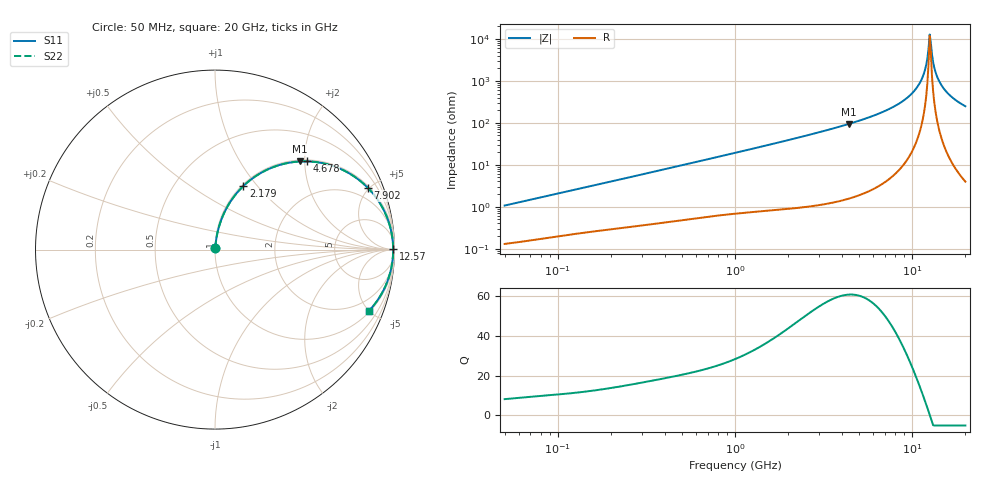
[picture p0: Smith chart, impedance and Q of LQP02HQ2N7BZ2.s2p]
!Murata Part Number: LQP02HQ2N7BZ2
!These Parameters are Measured in Series Mode Connection
!  o--[Z]--o
!Port1  Port2
!  o-------o
!Freq. Start=50[MHz] Stop=20[GHz], 401[Steps]
# Hz S RI R 50
!Freq.(Hz) S11(Real) S11(Imag) S21(Real) S21(Imag) S12(Real) S12(Imag) S22(Real) S22(Imag)
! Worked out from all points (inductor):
!   401 points, 50 MHz to 20 GHz, reference 50 ohm
!   read as one part in series: L = 3.34 nH near 51.52 MHz
!   highest Q = 60.5 at 4.406 GHz (marker M1), where L = 3.41 nH
!   self-resonance near 12.57 GHz
!   S11 on the Smith chart (normalised r, x): 50 MHz: 1.00, +0.02; 2.179 GHz: 1.02, +0.85; 4.678 GHz: 1.03, +2.04; 7.902 GHz: 1.11, +4.89; 12.57 GHz: open; 20 GHz: 1.08, -4.97
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5e7  0.00141 0.0105  0.9986 -0.0105  0.9986 -0.0105  0.00141 0.0105
1.364002e8  0.00311 0.0275  0.9969 -0.0275  0.9969 -0.0275  0.00311 0.0275
3.721004e8  0.00922 0.0718  0.9908 -0.0718  0.9908 -0.0718  0.00922 0.0718
1e9  0.0416 0.1826  0.9584 -0.1826  0.9584 -0.1826  0.0416 0.1826
2.179053e9  0.1577 0.3538  0.8423 -0.3538  0.8423 -0.3538  0.1577 0.3538
2.728004e9  0.2298 0.4112  0.7702 -0.4112  0.7702 -0.4112  0.2298 0.4112
4.405649e9  0.4719 0.491  0.5281 -0.491  0.5281 -0.491  0.4719 0.491
4.677679e9  0.5101 0.4917  0.4899 -0.4917  0.4899 -0.4917  0.5101 0.4917
7.442007e9  0.8166 0.3765  0.1834 -0.3765  0.1834 -0.3765  0.8166 0.3765
7.901521e9  0.8511 0.3446  0.1489 -0.3446  0.1489 -0.3446  0.8511 0.3446
9.457416e9  0.9359 0.2284  0.0641 -0.2284  0.0641 -0.2284  0.9359 0.2284
1.082228e10  0.9761 0.1255  0.0239 -0.1255  0.0239 -0.1255  0.9761 0.1255
1.166392e10  0.9883 0.0648  0.0117 -0.0648  0.0117 -0.0648  0.9883 0.0648
1.201863e10  0.991 0.04  0.009 -0.04  0.009 -0.04  0.991 0.04
1.238412e10  0.9925 0.0152  0.00752 -0.0152  0.00752 -0.0152  0.9925 0.0152
1.257102e10  0.9927 0.00277  0.00725 -0.00277  0.00725 -0.00277  0.9927 0.00277
1.295331e10  0.9923 -0.0221  0.00766 0.0221  0.00766 0.0221  0.9923 -0.0221
1.334722e10  0.9907 -0.047  0.00931 0.047  0.00931 0.047  0.9907 -0.047
1.375312e10  0.9878 -0.0717  0.0122 0.0717  0.0122 0.0717  0.9878 -0.0717
1.460232e10  0.9783 -0.1204  0.0217 0.1204  0.0217 0.1204  0.9783 -0.1204
1.670968e10  0.9398 -0.2243  0.0602 0.2243  0.0602 0.2243  0.9398 -0.2243
2e10  0.8565 -0.3427  0.1435 0.3427  0.1435 0.3427  0.8565 -0.3427
